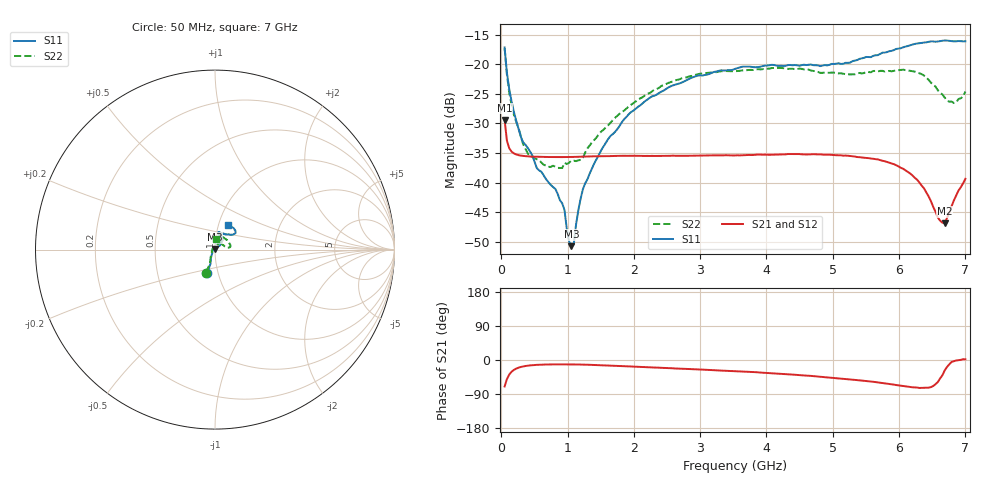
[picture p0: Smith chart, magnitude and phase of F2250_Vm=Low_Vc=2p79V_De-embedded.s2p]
! Integrated Device Technology
! Corporate Headquarters
! 6024 Silver Creek Valley Road
! San Jose, CA 95138  USA
! Phone:  1-408-284-8200
! Toll Free:  1-800-223-1366
! Webpage:  http://www.idt.com/
! Timing and RF Division
! 515 Groton Road, Suite 102
! Westford, MA 01886-6024
! Device:  F2250
! Description: Voltage Variable RF Attenuator
! Frequency:  50.0 -  6000.00 MHz
! Package:  3x3 mm Thin QFN Plastic Package: 16 pin
! Ports:  2 RF, 3 DC
!  Pin  1  = GND
!  Pin  2  = NC
!  Pin  3  = RF1  = Port 1
!  Pin  4  = NC
!  Pin  5  = GND
!  Pin  6  = GND
!  Pin  7  = GND
!  Pin  8  = GND
!  Pin  9  = NC
!  Pin 10  = RF2  = Port 2
!  Pin 11  = NC
!  Pin 12  = GND
!  Pin 13  = GND
!  Pin 14  = VCNTRL
!  Pin 15  = VDD
!  Pin 16  = VMODE
! Vcntrl:  2.790 Volts
! Vmode:  +0.000 Volts
! Vdd:  +3.30  Volts
! Current:  1.175 mA
! Data:  The device was measured on a the F2250 evaluation board which has
!  individual transmission lines to the RF pins.  Data was collected
!  using a calibrated network analyzer.  The evaluation board was
!  de-embedded using a TRL calibration technique.
!  The reference plane is the edge of the package pin.
! Misc:  SN 10
!  Action Tracker AT0258
! Date Measured:  2014-11-26
! Date:  2015-10-15  MJV
! Note:
!  Integrated Device Technology supplies this data as a sample of measured
!  data at the package pin for this product.  Your particular data for this
!  product may vary.
!  Data was taken at 25 degrees C.
!  Integrated Device Technology reserves the right to change this data at anytime.
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# GHz S dB R 50
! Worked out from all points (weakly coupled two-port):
!   201 points, 50 MHz to 7 GHz, reference 50 ohm
!   highest |S21| = -29.41 dB at 50 MHz (marker M1); lowest = -46.9 dB at 6.687 GHz (marker M2)
!   lowest |S11| = -50.7 dB at 1.058 GHz (marker M3), VSWR 1.01, Z = 49.8 + j0.242 ohm
!   |S11| at or under -10 dB: start of sweep to end of sweep
!   |S22| runs from -37.5 to -17.3 dB; largest |S21 - S12| = 7e-05
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0.05  -17.18 -108.6  -29.41 -69.8  -29.41 -69.8  -17.27 -111.0
0.08475  -21.45 -107.5  -32.92 -50.3  -32.92 -50.3  -21.74 -110.2
0.15425  -26.23 -116.6  -34.76 -31.1  -34.75 -31.1  -26.81 -122.5
0.29325  -32.21 -127.8  -35.43 -18.5  -35.43 -18.5  -32.09 -137.4
0.3975  -34.10 -141.8  -35.56 -15.0  -35.56 -15.0  -35.03 -160.3
0.5365  -37.57 -155.5  -35.64 -12.8  -35.63 -12.8  -36.05 178.0
0.91875  -43.50 157.7  -35.69 -11.5  -35.68 -11.5  -37.53 133.5
0.9535  -44.62 170.1  -35.68 -11.5  -35.69 -11.5  -36.65 131.1
1.023  -49.95 143.5  -35.68 -11.6  -35.67 -11.6  -36.63 116.0
1.05775  -50.73 123.5  -35.67 -11.6  -35.67 -11.6  -36.28 110.7
1.0925  -50.44 89.7  -35.66 -11.7  -35.66 -11.7  -36.29 106.3
1.162  -44.66 57.2  -35.64 -11.9  -35.64 -11.9  -36.22 95.6
1.2315  -41.09 44.3  -35.61 -12.1  -35.61 -12.1  -35.79 85.9
1.6485  -32.10 42.0  -35.52 -14.6  -35.51 -14.7  -29.88 64.5
2.37825  -24.87 47.4  -35.48 -20.3  -35.48 -20.3  -23.99 56.8
3.525  -20.79 72.4  -35.41 -29.5  -35.40 -29.5  -21.19 74.7
4.7065  -20.17 72.3  -35.19 -42.6  -35.20 -42.6  -21.14 72.3
5.85325  -17.81 40.5  -36.64 -63.3  -36.64 -63.4  -21.14 23.1
6.27025  -16.51 40.0  -39.49 -72.7  -39.50 -72.8  -21.36 9.7
6.68725  -15.99 48.8  -46.87 -27.7  -46.87 -27.3  -25.63 28.6
6.861  -16.13 55.1  -42.19 -1.3  -42.14 -1.3  -26.46 57.9
7  -16.13 63.2  -39.36 1.9  -39.31 1.8  -24.62 83.1
